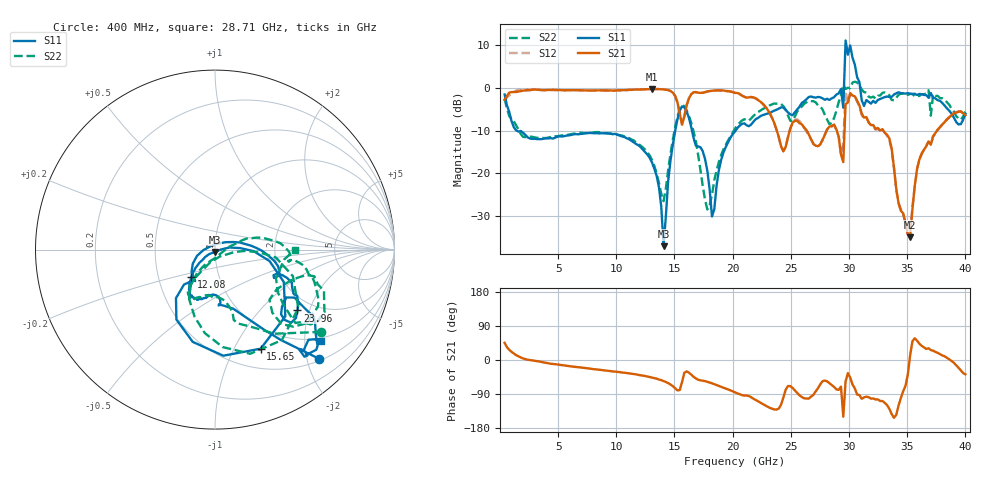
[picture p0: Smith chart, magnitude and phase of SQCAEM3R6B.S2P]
! Network Analyzer HP8722ES.07.66: Jul 25, 2000 Serial No. US39175408
! 26 Oct 2004  14:10:07
! Frequency  S11  S21  S12  S22
# HZ  S  DB R  50
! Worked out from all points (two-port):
!   201 points, 400 MHz to 40 GHz, reference 50 ohm
!   highest |S21| = -0.26 dB at 13.07 GHz (marker M1); lowest = -35.1 dB at 35.25 GHz (marker M2)
!   |S21| within 3 dB of the highest: start of sweep to 15.24 GHz; 16.14 GHz to 22.39 GHz (6.249 GHz wide, 32.4 % of centre)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
!   lowest |S11| = -37.2 dB at 14.06 GHz (marker M3), VSWR 1.03, Z = 49.8 - j1.36 ohm
!   |S11| at or under -10 dB: 1.416 GHz to 15.06 GHz (13.65 GHz wide, 166 % of centre); 16.5 GHz to 20.26 GHz (3.755 GHz wide, 20.4 % of centre)
!   |S22| runs from -28.5 to 1.5 dB; largest |S21 - S12| = 0.34
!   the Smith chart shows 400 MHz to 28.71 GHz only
!   S11 on the Smith chart (normalised r, x): 400 MHz: 0.54, -2.22; 12.08 GHz: 0.73, -0.23; 15.65 GHz: 0.73, -1.28; 23.96 GHz: 1.66, -1.67; 28.71 GHz: 0.92, -2.38
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4e8  -1.54 -46.4  -2.79 45.2  -3.01 50.3  -2.52 -37.8
7.132e9  -10.76 -108.4  -0.56 -20.4  -0.59 -20.8  -10.60 -113.4
1.2082e10  -13.88 -130.9  -0.37 -40.2  -0.33 -39.9  -13.52 -125.0
1.3072e10  -17.53 -137.8  -0.26 -46.4  -0.29 -46.2  -16.94 -122.3
1.3666e10  -23.36 -143.2  -0.27 -51.5  -0.26 -51.0  -22.33 -110.4
1.4062e10  -37.16 -98.5  -0.32 -55.5  -0.33 -55.1  -26.59 -56.8
1.5646e10  -4.32 -65.2  -8.60 -58.7  -8.62 -57.2  -4.05 -53.6
1.822e10  -30.19 143.0  -0.67 -61.4  -0.59 -61.2  -25.11 -3.3
2.02e10  -10.22 -7.6  -1.18 -85.4  -1.06 -84.4  -9.57 8.5
2.3962e10  -4.87 -36.4  -11.52 -128.0  -11.66 -127.6  -3.71 -36.2
2.6932e10  -2.19 -48.7  -13.17 -92.1  -13.03 -91.3  -3.11 -34.7
2.8714e10  -2.17 -40.9  -8.62 -71.0  -8.64 -71.1  -7.04 -0.3
2.9506e10  -4.64 23.7  -17.42 -149.7  -13.10 -124.7  0.75 32.9
2.9704e10  11.15 -52.3  -3.78 -56.5  -0.80 -41.0  -0.24 -64.4
3.01e10  9.97 -69.7  -1.21 -46.1  -1.37 -46.3  -0.04 -11.5
3.0496e10  5.50 -83.3  -1.96 -74.6  -1.88 -74.1  1.47 -37.5
3.0694e10  2.52 84.8  -3.00 -91.3  -3.17 -90.7  1.28 133.2
3.1288e10  -4.24 99.6  -6.94 -98.6  -7.23 -99.8  -0.99 127.5
3.1486e10  -2.84 -69.5  -6.87 -96.8  -6.94 -98.1  -1.07 -53.2
3.3466e10  -2.12 -46.9  -11.87 -128.9  -12.22 -128.2  -1.73 -47.3
3.5248e10  -1.34 -61.1  -35.11 11.5  -34.12 11.8  -1.40 -31.4
4e10  -6.09 -51.1  -6.41 -37.9  -6.54 -37.2  -5.52 -3.8
